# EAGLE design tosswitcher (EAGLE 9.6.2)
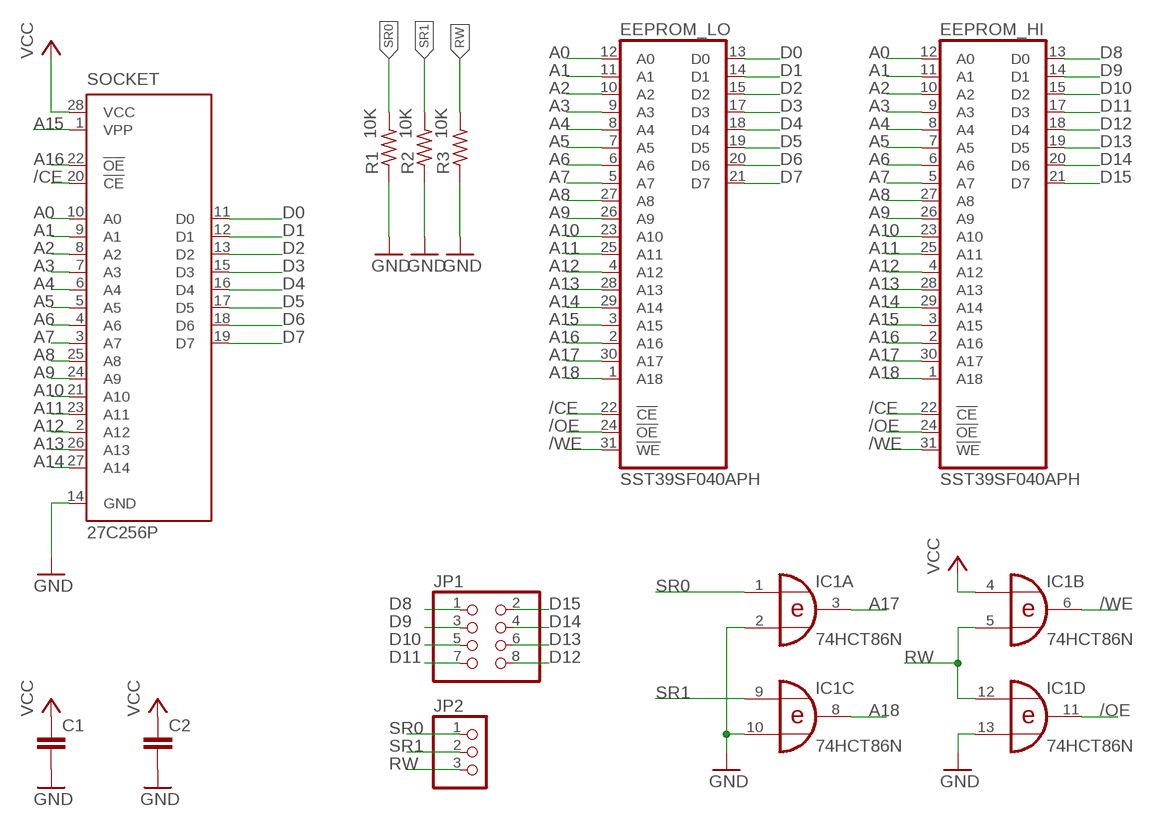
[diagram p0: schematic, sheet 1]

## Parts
C1  C2,5-3  [C2.5-3]
C2  C2,5-3  [C2.5-3]
EEPROM_HI  SST39SF040APH  [DIL32]
EEPROM_LO  SST39SF040APH  [DIL32]
IC1  74HCT86N  [DIL14]
JP1  PINHD-2X4/90  [2X04/90]
JP2  PINHD-1X3/90  [1X03/90]
R1  10K  R-US_0204/5  [0204/5]
R2  10K  R-US_0204/7  [0204/7]
R3  10K  R-US_0204/7  [0204/7]
SOCKET  27C256P  [DIL28-6]

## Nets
/CE: EEPROM_HI.22(!CE) EEPROM_LO.22(!CE) SOCKET.20(!CE)
/OE: EEPROM_HI.24(!OE) EEPROM_LO.24(!OE) IC1.11(D:O)
/WE: EEPROM_HI.31(!WE) EEPROM_LO.31(!WE) IC1.6(B:O)
A0: EEPROM_HI.12(A0) EEPROM_LO.12(A0) SOCKET.10(A0)
A1: EEPROM_HI.11(A1) EEPROM_LO.11(A1) SOCKET.9(A1)
A2: EEPROM_HI.10(A2) EEPROM_LO.10(A2) SOCKET.8(A2)
A3: EEPROM_HI.9(A3) EEPROM_LO.9(A3) SOCKET.7(A3)
A4: EEPROM_HI.8(A4) EEPROM_LO.8(A4) SOCKET.6(A4)
A5: EEPROM_HI.7(A5) EEPROM_LO.7(A5) SOCKET.5(A5)
A6: EEPROM_HI.6(A6) EEPROM_LO.6(A6) SOCKET.4(A6)
A7: EEPROM_HI.5(A7) EEPROM_LO.5(A7) SOCKET.3(A7)
A8: EEPROM_HI.27(A8) EEPROM_LO.27(A8) SOCKET.25(A8)
A9: EEPROM_HI.26(A9) EEPROM_LO.26(A9) SOCKET.24(A9)
A10: EEPROM_HI.23(A10) EEPROM_LO.23(A10) SOCKET.21(A10)
A11: EEPROM_HI.25(A11) EEPROM_LO.25(A11) SOCKET.23(A11)
A12: EEPROM_HI.4(A12) EEPROM_LO.4(A12) SOCKET.2(A12)
A13: EEPROM_HI.28(A13) EEPROM_LO.28(A13) SOCKET.26(A13)
A14: EEPROM_HI.29(A14) EEPROM_LO.29(A14) SOCKET.27(A14)
A15: EEPROM_HI.3(A15) EEPROM_LO.3(A15) SOCKET.1(VPP)
A16: EEPROM_HI.2(A16) EEPROM_LO.2(A16) SOCKET.22(!OE)
A17: EEPROM_HI.30(A17) EEPROM_LO.30(A17) IC1.3(A:O)
A18: EEPROM_HI.1(A18) EEPROM_LO.1(A18) IC1.8(C:O)
D0: EEPROM_LO.13(D0) SOCKET.11(D0)
D1: EEPROM_LO.14(D1) SOCKET.12(D1)
D2: EEPROM_LO.15(D2) SOCKET.13(D2)
D3: EEPROM_LO.17(D3) SOCKET.15(D3)
D4: EEPROM_LO.18(D4) SOCKET.16(D4)
D5: EEPROM_LO.19(D5) SOCKET.17(D5)
D6: EEPROM_LO.20(D6) SOCKET.18(D6)
D7: EEPROM_LO.21(D7) SOCKET.19(D7)
D8: EEPROM_HI.13(D0) JP1.1
D9: EEPROM_HI.14(D1) JP1.3
D10: EEPROM_HI.15(D2) JP1.5
D11: EEPROM_HI.17(D3) JP1.7
D12: EEPROM_HI.18(D4) JP1.8
D13: EEPROM_HI.19(D5) JP1.6
D14: EEPROM_HI.20(D6) JP1.4
D15: EEPROM_HI.21(D7) JP1.2
GND: C1.2 C2.2 IC1.2(A:I1) IC1.10(C:I1) IC1.13(D:I1) R1.1 R2.1 R3.1 SOCKET.14(GND)
RW: IC1.5(B:I1) IC1.12(D:I0) JP2.3 R3.2
SR0: IC1.1(A:I0) JP2.1 R1.2
SR1: IC1.9(C:I0) JP2.2 R2.2
VCC: C1.1 C2.1 IC1.4(B:I0) SOCKET.28(VCC)

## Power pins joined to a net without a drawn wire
GND: EEPROM_HI.16(GND) EEPROM_LO.16(GND) IC1.7(P:GND)
VCC: EEPROM_HI.32(VCC) EEPROM_LO.32(VCC) IC1.14(P:VCC)

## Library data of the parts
C1 C2 = capacitor-wima:C: CAPACITOR
EEPROM_HI EEPROM_LO = SST39SF040:SST39SF040A: 4 Mbit x8 Multi-Purpose Flash Source: http://www.sst.com/dotAsset/40782.pdf
IC1 = 74xx-eu:74*86: Quad 2-input EXCLUSIVE-OR (XOR) gate
JP1 = pinhead:PINHD-2X4: PIN HEADER
JP2 = pinhead:PINHD-1X3: PIN HEADER
R1-R3 = rcl:R-US_: RESISTOR, American symbol; SPICEPREFIX: R
SOCKET = socket:27*256: CMOS EPROM 256 K (32 K x 8), low voltage; MF: Arrow Electronics; MPN: M27C256B15F1; OC_FARNELL: 1125431; OC_NEWARK: 93K7335

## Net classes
0 default: clearance 0.205 mm

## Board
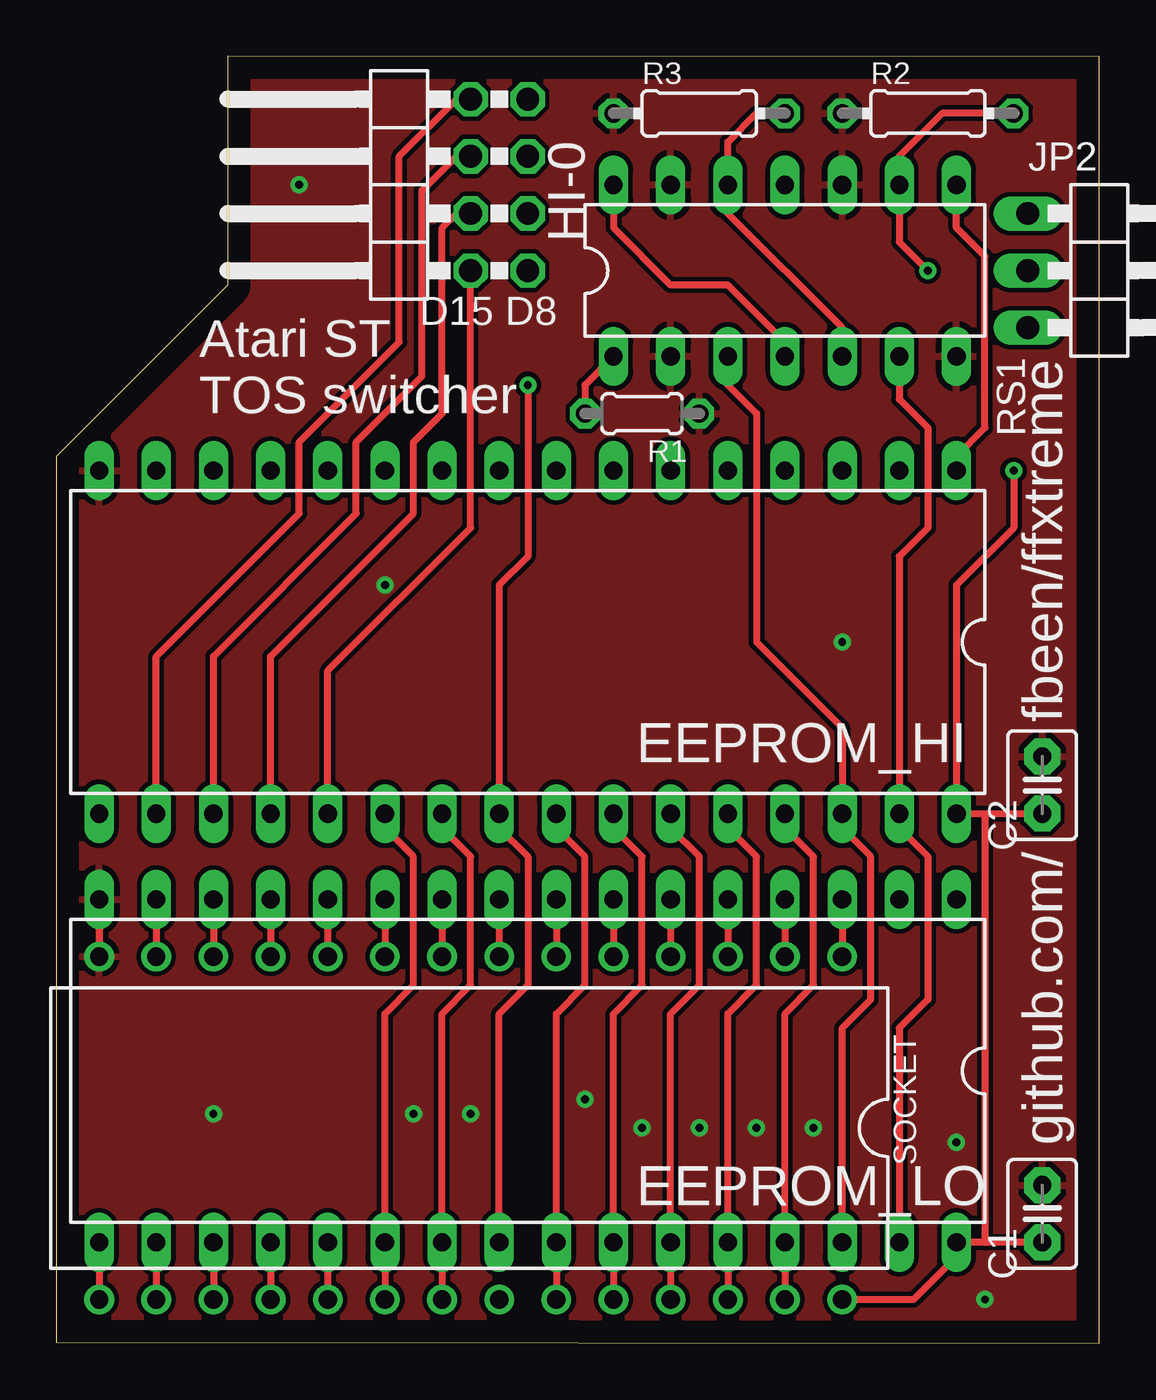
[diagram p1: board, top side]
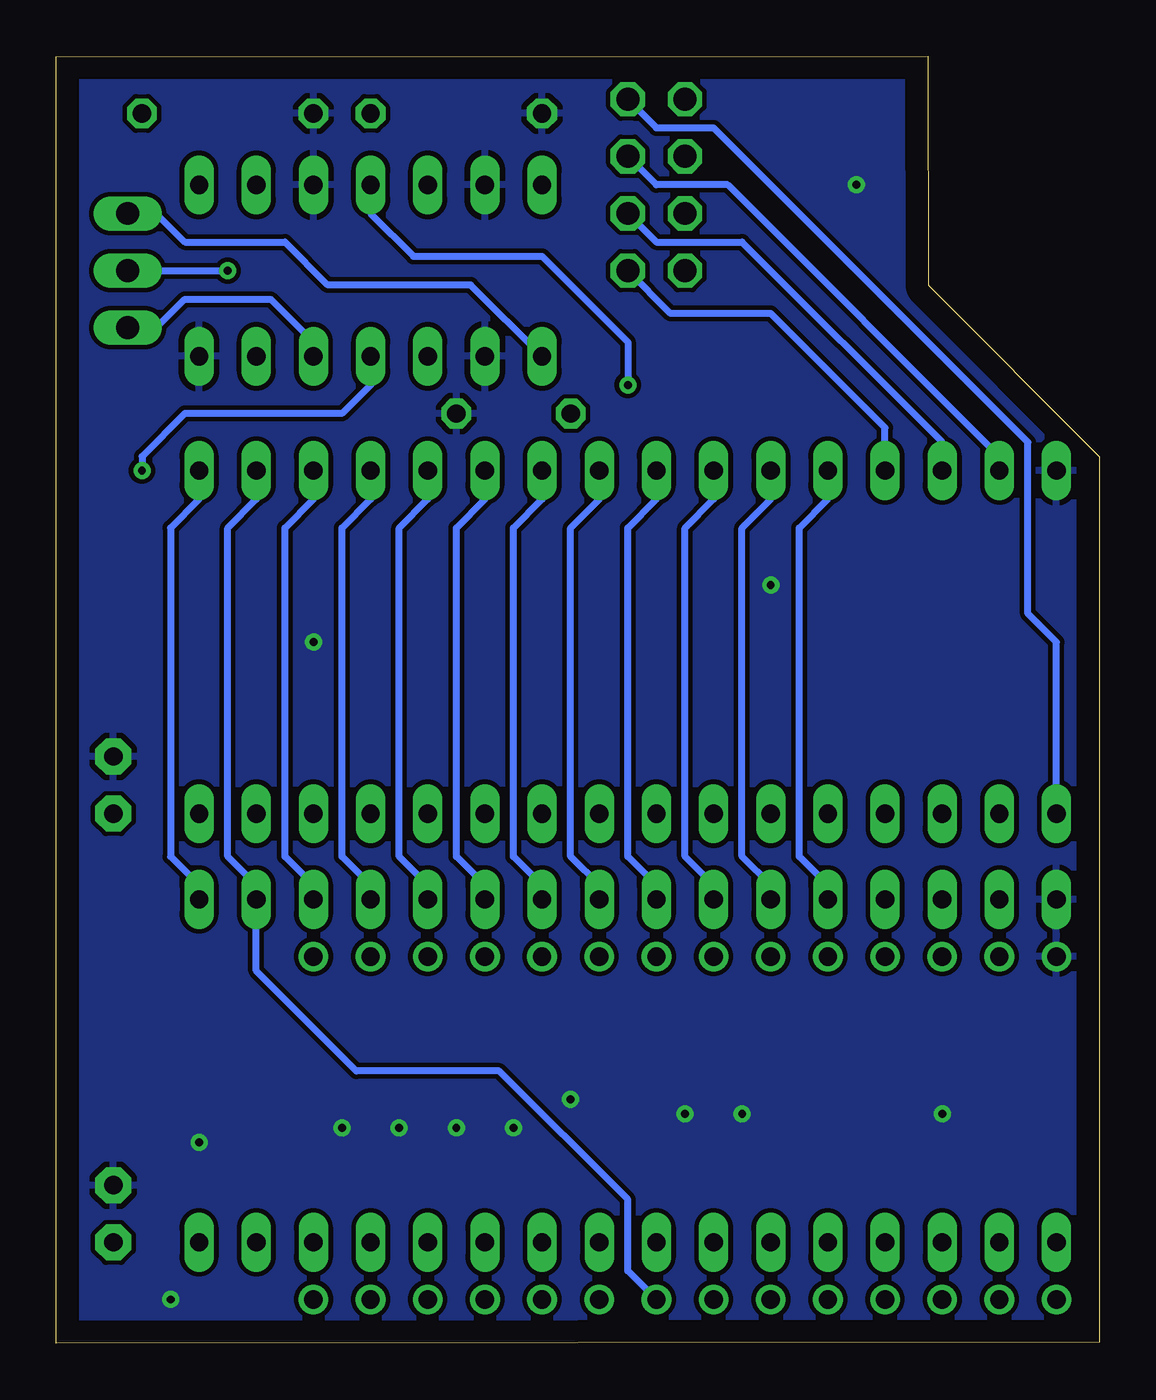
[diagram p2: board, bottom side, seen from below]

Size 46.35 x 57.19 mm. Coordinates in mm from the lower left corner, seen from the top.
Outline: 0,0.04 46.35,0 46.35,57.16 7.62,57.19 7.61,47.02 0,39.4 0,0.04
Copper layers (1*16): Top 0.035mm / dielectric 1.5mm / Bottom 0.035mm
Design rules "default": minimum track width 6mil, minimum drill 0.35mm, track to track 6mil, track to pad 6mil, pad to pad 6mil, via to via 6mil, smd to smd 6mil, copper to edge 40mil, drill to drill 6mil, minimum pad ring 10mil, minimum via ring 8mil, stop-mask expansion 4mil, vias tented up to drill 0mil, thermal gap 10mil

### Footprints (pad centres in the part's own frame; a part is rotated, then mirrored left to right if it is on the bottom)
C2.5-3 = drill 0.813 pad 1.6 octagon: 1 -1.27,0; 2 1.27,0
DIL32 = drill 0.813 long: 1 -19.05,-7.62; 2 -16.51,-7.62; 3 -13.97,-7.62; 4 -11.43,-7.62; 5 -8.89,-7.62; 6 -6.35,-7.62; 7 -3.81,-7.62; 8 -1.27,-7.62; 9 1.27,-7.62; 10 3.81,-7.62; 11 6.35,-7.62; 12 8.89,-7.62; 13 11.43,-7.62; 14 13.97,-7.62; 15 16.51,-7.62; 16 19.05,-7.62; 17 19.05,7.62; 18 16.51,7.62; 19 13.97,7.62; 20 11.43,7.62; 21 8.89,7.62; 22 6.35,7.62; 23 3.81,7.62; 24 1.27,7.62; 25 -1.27,7.62; 26 -3.81,7.62; 27 -6.35,7.62; 28 -8.89,7.62; 29 -11.43,7.62; 30 -13.97,7.62; 31 -16.51,7.62; 32 -19.05,7.62
DIL14 = drill 0.813 long: 1 -7.62,-3.81; 2 -5.08,-3.81; 3 -2.54,-3.81; 4 0,-3.81; 5 2.54,-3.81; 6 5.08,-3.81; 7 7.62,-3.81; 8 7.62,3.81; 9 5.08,3.81; 10 2.54,3.81; 11 0,3.81; 12 -2.54,3.81; 13 -5.08,3.81; 14 -7.62,3.81
2X04/90 = drill 1.016 octagon: 1 -3.81,-6.35; 2 -3.81,-3.81; 3 -1.27,-6.35; 4 -1.27,-3.81; 5 1.27,-6.35; 6 1.27,-3.81; 7 3.81,-6.35; 8 3.81,-3.81
1X03/90 = drill 1.016 long: 1 -2.54,-3.81; 2 0,-3.81; 3 2.54,-3.81
0204/5 = drill 0.813 octagon: 1 -2.54,0; 2 2.54,0
0204/7 = drill 0.813 octagon: 1 -3.81,0; 2 3.81,0
DIL28-6 = drill 0.813: 1 -16.51,-7.62; 2 -13.97,-7.62; 3 -11.43,-7.62; 4 -8.89,-7.62; 5 -6.35,-7.62; 6 -3.81,-7.62; 7 -1.27,-7.62; 8 1.27,-7.62; 9 3.81,-7.62; 10 6.35,-7.62; 11 8.89,-7.62; 12 11.43,-7.62; 13 13.97,-7.62; 14 16.51,-7.62; 15 16.51,7.62; 16 13.97,7.62; 17 11.43,7.62; 18 8.89,7.62; 19 6.35,7.62; 20 3.81,7.62; 21 1.27,7.62; 22 -1.27,7.62; 23 -3.81,7.62; 24 -6.35,7.62; 25 -8.89,7.62; 26 -11.43,7.62; 27 -13.97,7.62; 28 -16.51,7.62

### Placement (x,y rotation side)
C1  43.81,5.75 90 top
C2  43.81,24.8 90 top
EEPROM_HI  20.95,31.15 180 top
EEPROM_LO  20.95,12.1 180 top
IC1  32.38,47.66 0 top
JP1  14.61,51.47 90 top
JP2  46.99,47.66 270 top
R1  26.04,41.31 180 top
R2  38.73,54.65 0 top
R3  28.57,54.65 0 top
SOCKET  18.41,9.56 180 top

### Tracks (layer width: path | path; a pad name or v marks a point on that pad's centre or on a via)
/CE
  Top 0.305: SOCKET.20 EEPROM_LO.22 14.61,14.64 15.88,15.91 15.88,21.63 14.61,22.9 EEPROM_HI.22
/OE  (via drill 0.35)
  Top 0.305: v20.95,42.58 20.95,34.96 19.68,33.69 EEPROM_HI.24 19.68,22.9 20.95,21.63 20.95,15.91 19.68,14.64 EEPROM_LO.24
  Bottom 0.305: IC1.11 32.38,50.2 30.48,48.3 24.77,48.3 20.95,44.49 v20.95,42.58
/WE
  Top 0.305: IC1.6 37.47,41.95 38.73,40.68 38.73,36.23 37.47,34.96 EEPROM_HI.31 37.47,22.9 38.73,21.63 38.73,15.28 37.47,14.01 EEPROM_LO.31
A0
  Top 0.305: EEPROM_LO.12 SOCKET.10
  Bottom 0.305: EEPROM_LO.12 12.06,20.36 13.34,21.63 13.34,36.23 12.06,37.5 EEPROM_HI.12
A1
  Top 0.305: EEPROM_LO.11 SOCKET.9
  Bottom 0.305: EEPROM_LO.11 14.61,20.36 15.88,21.63 15.88,36.23 14.61,37.5 EEPROM_HI.11
A2
  Top 0.305: EEPROM_LO.10 SOCKET.8
  Bottom 0.305: EEPROM_LO.10 17.14,20.36 18.41,21.63 18.41,36.23 17.14,37.5 EEPROM_HI.10
A3
  Top 0.305: EEPROM_LO.9 SOCKET.7
  Bottom 0.305: EEPROM_LO.9 19.68,20.36 20.95,21.63 20.95,36.23 19.68,37.5 EEPROM_HI.9
A4
  Top 0.305: EEPROM_LO.8 SOCKET.6
  Bottom 0.305: EEPROM_LO.8 22.23,20.36 23.5,21.63 23.5,36.23 22.23,37.5 EEPROM_HI.8
A5
  Top 0.305: EEPROM_LO.7 SOCKET.5
  Bottom 0.305: EEPROM_LO.7 24.77,20.36 26.04,21.63 26.04,36.23 24.77,37.5 EEPROM_HI.7
A6
  Top 0.305: EEPROM_LO.6 SOCKET.4
  Bottom 0.305: EEPROM_LO.6 27.3,20.36 28.57,21.63 28.57,36.23 27.3,37.5 EEPROM_HI.6
A7
  Top 0.305: EEPROM_LO.5 SOCKET.3
  Bottom 0.305: EEPROM_LO.5 29.84,20.36 31.11,21.63 31.11,36.23 29.84,37.5 EEPROM_HI.5
A8
  Top 0.305: SOCKET.25 EEPROM_LO.27 27.3,14.64 28.57,15.91 28.57,21.63 27.3,22.9 EEPROM_HI.27
A9
  Top 0.305: SOCKET.24 EEPROM_LO.26 24.77,14.64 26.04,15.91 26.04,21.63 24.77,22.9 EEPROM_HI.26
A10
  Top 0.305: SOCKET.21 EEPROM_LO.23 17.14,14.64 18.41,15.91 18.41,21.63 17.14,22.9 EEPROM_HI.23
A11
  Top 0.305: SOCKET.23 EEPROM_LO.25 22.23,14.64 23.5,15.91 23.5,21.63 22.23,22.9 EEPROM_HI.25
A12
  Top 0.305: EEPROM_LO.4 SOCKET.2
  Bottom 0.305: EEPROM_LO.4 32.38,20.36 33.66,21.63 33.66,36.23 32.38,37.5 EEPROM_HI.4
A13
  Top 0.305: SOCKET.26 EEPROM_LO.28 29.84,14.64 31.11,15.91 31.11,21.63 29.84,22.9 EEPROM_HI.28
A14
  Top 0.305: SOCKET.27 EEPROM_LO.29 32.38,14.64 33.66,15.91 33.66,21.63 32.38,22.9 EEPROM_HI.29
A15
  Top 0.305: EEPROM_LO.3 SOCKET.1
  Bottom 0.305: EEPROM_LO.3 34.92,20.36 36.2,21.63 36.2,36.23 34.92,37.5 EEPROM_HI.3
A16
  Bottom 0.305: SOCKET.22 20.95,3.21 20.95,6.39 26.67,12.1 33.02,12.1 37.47,16.55 EEPROM_LO.2 37.47,20.36 38.73,21.63 38.73,36.23 37.47,37.5 EEPROM_HI.2
A17
  Top 0.305: EEPROM_LO.30 34.92,14.01 36.2,15.28 36.2,21.63 34.92,22.9 EEPROM_HI.30 34.92,27.34 31.11,31.15 31.11,41.31 29.84,42.58 IC1.3
A18
  Top 0.305: EEPROM_HI.1 40.01,39.41 41.27,40.68 41.27,48.3 40.01,49.57 IC1.8
  Bottom 0.305: EEPROM_HI.1 40.01,37.5 41.27,36.23 41.27,21.63 40.01,20.36 EEPROM_LO.1
D0
  Top 0.305: EEPROM_LO.13 SOCKET.11
D1
  Top 0.305: EEPROM_LO.14 SOCKET.12
D2
  Top 0.305: EEPROM_LO.15 SOCKET.13
D3
  Top 0.305: EEPROM_LO.17 SOCKET.15
D4
  Top 0.305: EEPROM_LO.18 SOCKET.16
D5
  Top 0.305: EEPROM_LO.19 SOCKET.17
D6
  Top 0.305: EEPROM_LO.20 SOCKET.18
D7
  Top 0.305: EEPROM_LO.21 SOCKET.19
D8
  Bottom 0.305: EEPROM_HI.13 9.53,40.68 14.61,45.76 19.05,45.76 JP1.1
D9
  Bottom 0.305: EEPROM_HI.14 6.99,40.04 15.88,48.93 19.68,48.93 JP1.3
D10
  Bottom 0.305: EEPROM_HI.15 4.45,39.41 16.51,51.47 19.68,51.47 JP1.5
D11
  Bottom 0.305: EEPROM_HI.17 1.91,31.15 3.17,32.42 3.17,40.04 17.14,54.01 19.68,54.01 JP1.7
D12
  Top 0.305: EEPROM_HI.18 4.45,30.52 10.79,36.87 10.79,40.04 15.24,44.49 15.24,52.74 17.78,55.28 JP1.8
D13
  Top 0.305: EEPROM_HI.19 6.99,30.52 13.34,36.87 13.34,40.04 16.26,42.96 16.26,51.22 17.78,52.74 JP1.6
D14
  Top 0.305: EEPROM_HI.20 9.53,30.52 15.88,36.87 15.88,40.04 17.14,41.31 17.14,49.57 17.78,50.2 JP1.4
D15
  Top 0.305: EEPROM_HI.21 12.06,29.88 18.41,36.23 JP1.2
GND  (via drill 0.35)
  Top 0.305: EEPROM_LO.16 SOCKET.14
  other vias: 40.01,8.93 41.27,1.94 6.99,10.2 18.41,10.2 15.88,10.2 23.5,10.83 26.04,9.56 28.57,9.56 31.11,9.56 33.66,9.56 14.61,33.69 34.92,31.15 10.79,51.47
  pour Top: 7.62,57.19 46.35,57.19 46.35,0.04 0,0.04 0,39.41 7.62,47.03
  pour Bottom: 7.62,57.19 46.35,57.19 46.35,0.04 0,0.04 0,39.41 7.62,47.03
RW
  Top 0.305: R3.2 31.11,54.65 29.84,53.38 IC1.12 29.84,50.2 34.92,45.12 IC1.5
  Bottom 0.305: JP2.3 41.91,45.12 40.64,46.39 36.83,46.39 34.92,44.49 IC1.5
SR0
  Top 0.305: IC1.1 23.5,42.58 R1.2
  Bottom 0.305: IC1.1 27.94,47.03 34.29,47.03 36.2,48.93 40.64,48.93 41.91,50.2 JP2.1
SR1  (via drill 0.35)
  Top 0.305: v38.73,47.66 37.47,48.93 IC1.9 37.47,52.74 39.37,54.65 R2.2
  Bottom 0.305: JP2.2 v38.73,47.66
VCC  (via drill 0.35)
  Top 0.305: SOCKET.28 38.1,1.94 40.01,3.85 EEPROM_LO.32 41.27,4.48 | 41.27,23.53 EEPROM_HI.32 40.01,33.69 42.55,36.23 v42.55,38.77 | 41.27,23.53 C2.1 | C1.1 41.27,4.48 | 41.27,23.53 41.27,4.48 | IC1.14 24.77,49.57 27.3,47.03 29.84,47.03 32.38,44.49 IC1.4
  Bottom 0.305: v42.55,38.77 42.55,39.41 40.64,41.31 33.66,41.31 32.38,42.58 IC1.4

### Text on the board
tNames: HI-0 | D15 | D8 | Atari ST / TOS switcher | RS1 | fbeen/ffxtreme | github.com/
